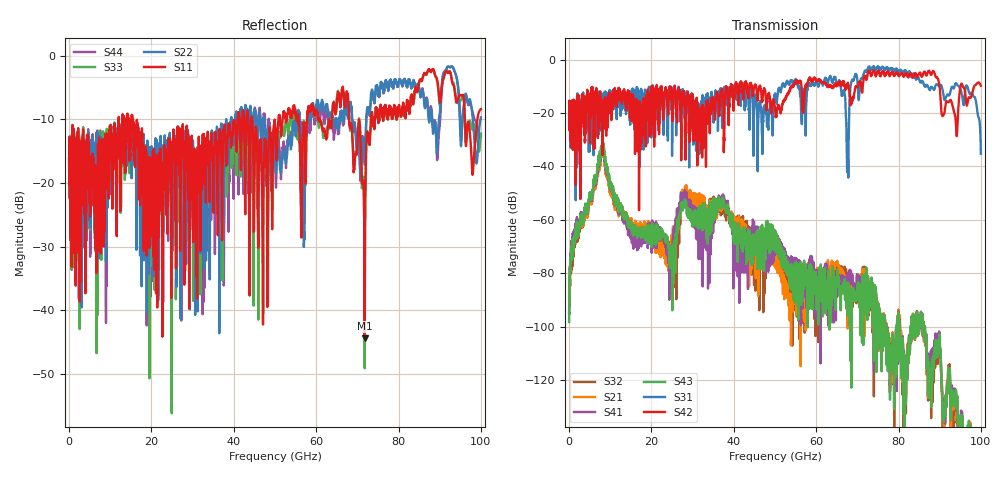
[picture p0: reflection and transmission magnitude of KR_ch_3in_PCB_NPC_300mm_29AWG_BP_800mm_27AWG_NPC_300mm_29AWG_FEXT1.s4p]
# GHz S RI R 45
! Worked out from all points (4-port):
!   4000 points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, 25 MHz to 100 GHz, reference 45 ohm
!   strongest paths, dB at 25 MHz, 25.02 GHz, 50.02 GHz, 75.03 GHz, 100 GHz:
!     S42: -20.6, -18.0, -18.0, -4.3, -9.8
!     S31: -20.6, -36.0, -12.7, -2.5, -35.2
!     S43: -98.2, -89.6, -66.0, -96.1, -142.5
!     S41: -95.2, -73.0, -67.7, -96.2, -143.8
!     S21: -88.9, -69.1, -77.1, -96.1, -148.9
!     S32: -94.9, -72.0, -74.9, -96.0, -147.8
!   lowest |S11| = -44.4 dB at 71.78 GHz (marker M1), VSWR 1.01, Z = 44.7 - j0.45 ohm
!   |S11| at or under -10 dB: start of sweep to 12.05 GHz; 15.53 GHz to 40.98 GHz (25.45 GHz wide, 90.1 % of centre); 44.43 GHz to 50.83 GHz (6.396 GHz wide, 13.4 % of centre)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
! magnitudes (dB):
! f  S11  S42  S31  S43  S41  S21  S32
! 25 MHz  -16.1  -20.6  -20.6  -98.2  -95.2  -88.9  -94.9
! 8.1 GHz  -26.7  -24.1  -18.9  -31.6  -32.8  -34.1  -32.8
! 24.43 GHz  -12.9  -11.2  -10.2  -74.7  -83.1  -81.0  -73.3
! 27.95 GHz  -20.2  -13.4  -19.2  -54.0  -51.3  -51.0  -52.5
! 67.6 GHz  -6.0  -9.9  -32.2  -87.2  -85.2  -89.0  -81.5
! 71.78 GHz  -44.4  -6.1  -4.3  -91.8  -89.8  -86.3  -85.4
! 100 GHz  -8.4  -9.8  -35.2  -142.5  -143.8  -148.9  -147.8
